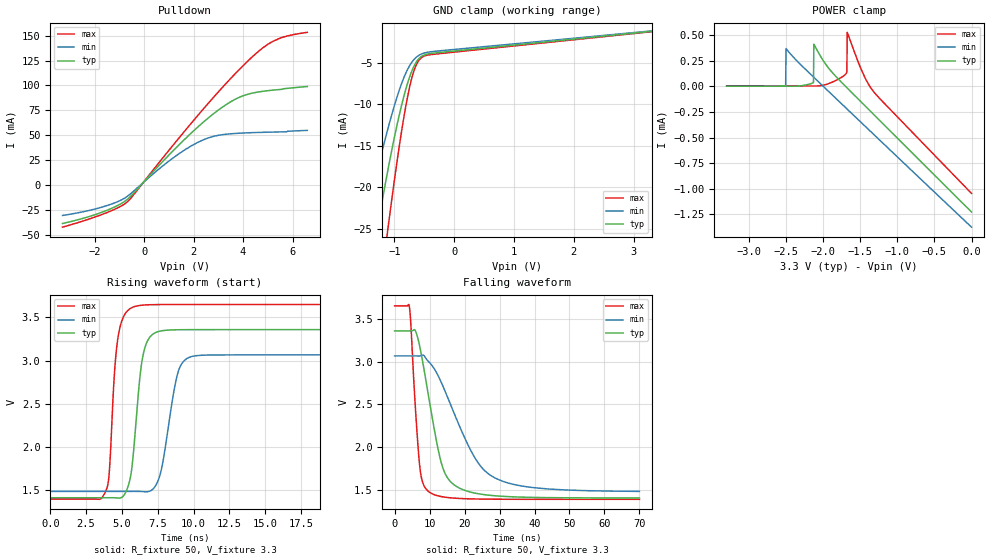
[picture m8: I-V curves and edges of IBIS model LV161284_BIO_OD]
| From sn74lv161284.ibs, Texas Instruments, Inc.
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[Model]   LV161284_BIO_OD
Model_type  I/O_open_drain
Vinl=0.8
Vinh=2.0
Enable   Active-High
Vref =   3.3
Rref =   500
Cref =   50p
Vmeas =   1.4
| variable   typ   min   max
C_comp   5.52pF   4.67pF   6.22pF
| C_pulldown   5.17pF   4.57pF   5.68pF
| C_tri-state   5.52pF   4.67pF   6.22pF
[Temperature Range]   40   100   -40
| Ambient temperature   25   85   -40
[Voltage range]   3.3   3   3.6
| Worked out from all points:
|   slope of the pulldown table from 0 to 0.495 V, typ, clamps not added: 37 ohm
|   rising waveform, R_fixture 50, V_fixture 3.3: 20-80 % time 652ps typ, 918ps min, 498ps max; typ from 1.41 V to 3.36 V
|   falling waveform, R_fixture 50, V_fixture 3.3: 20-80 % time 5.34ns typ, 10.8ns min, 2.07ns max; typ from 3.36 V to 1.41 V
[GND Clamp]
| LV161284_BIO_OD
|   Voltage   I(typ)   I(min)   I(max)
-3.3V     -132.9mA   -95.54mA   -170.5mA
-1.54V    -36.32mA   -26.12mA   -50.92mA
-1.495V   -34.24mA   -24.64mA   -48.09mA
-1.295V   -25.43mA   -18.32mA   -35.84mA
-1.275V   -24.59mA   -17.72mA   -34.65mA
-1.11V    -18mA      -13.01mA   -25.13mA
-920mV    -11.37mA   -8.353mA   -15.17mA
-785mV    -7.61mA    -5.896mA   -9.329mA
-675mV    -5.466mA   -4.642mA   -6.029mA
-560mV    -4.309mA   -3.992mA   -4.463mA
-370mV    -3.864mA   -3.66mA    -4.005mA
3.3V      -1.226mA   -1.168mA   -1.268mA
[POWER Clamp]
| LV161284_BIO_OD
|   Voltage   I(typ)   I(min)   I(max)
-3.3V     318.9nA    13.56nA    4.426uA
-2.505V   202.9nA    4.995uA    2.684uA
-2.5V     202.5nA    367uA      2.674uA
-2.13V    36.28uA    89.82uA    2.09uA
-2.125V   410uA      86.37uA    2.092uA
-1.94V    189.5uA    -41.39uA   21.68uA
-1.685V   -10.57uA   -217.2uA   128.8uA
-1.68V    -14.2uA    -220.7uA   137.3uA
-1.675V   -17.83uA   -224.1uA   525.1uA
-1.475V   -162.4uA   -361.8uA   145uA
-1.33V    -267.1uA   -461.6uA   -43.55uA
-48.03fV  -1.226mA   -1.373mA   -1.045mA
[Pulldown]
| LV161284_BIO_OD
|   Voltage   I(typ)   I(min)   I(max)
-3.3V     -38.49mA   -30.42mA   -42.13mA
-1.69V    -27.01mA   -21.92mA   -29.3mA
-1.045V   -20.07mA   -16.3mA    -22.51mA
-680mV    -14.27mA   -11.21mA   -16.75mA
810mV     25.23mA    20.41mA    29.02mA
1.84V     50.74mA    38.38mA    60.19mA
2.68V     69.12mA    48.05mA    84.54mA
3.58V     84.76mA    51.67mA    109.1mA
4.215V    91.3mA     52.52mA    125mA
5.08V     94.99mA    53.16mA    142.4mA
5.665V    96.78mA    53.47mA    148.8mA
6.6V      98.93mA    54.94mA    153.3mA
[Ramp]
| LV161284_BIO_OD
| variable   typ   min   max
dV/dt_r   1.17/6.60E-10   0.95/9.22E-10   1.36/5.00E-10
dV/dt_f   1.18/5.37E-09   0.95/1.08E-08   1.36/2.08E-09
R_load = 50
[Rising Waveform]
| LV161284_BIO_OD
R_fixture =   50
C_fixture =   0
L_fixture =   0
V_fixture =   3.3
V_fixture_min = 3
V_fixture_max = 3.6
|   Time   V(typ)   V(min)   V(max)
0s        1.409V     1.483V     1.393V
3.88ns    1.409V     1.483V     1.487V
4.75ns    1.406V     1.483V     3.29V
5.58ns    1.635V     1.483V     3.603V
6.1ns     2.521V     1.483V     3.635V
6.945ns   3.271V     1.485V     3.647V
7.735ns   3.344V     1.721V     3.649V
8.96ns    3.357V     2.886V     3.65V
10.11ns   3.358V     3.055V     3.65V
70ns      3.359V     3.066V     3.65V
[Falling Waveform]
| LV161284_BIO_OD
R_fixture =   50
C_fixture =   0
L_fixture =   0
V_fixture =   3.3
V_fixture_min = 3
V_fixture_max = 3.6
|   Time   V(typ)   V(min)   V(max)
0s        3.359V     3.066V     3.65V
4.205ns   3.359V     3.066V     3.645V
5.865ns   3.366V     3.066V     2.515V
7.155ns   3.184V     3.066V     1.791V
9.745ns   2.588V     2.999V     1.483V
13.82ns   1.757V     2.713V     1.422V
18.72ns   1.52V      2.232V     1.403V
24.55ns   1.454V     1.782V     1.397V
31.04ns   1.428V     1.602V     1.394V
70ns      1.409V     1.486V     1.393V
